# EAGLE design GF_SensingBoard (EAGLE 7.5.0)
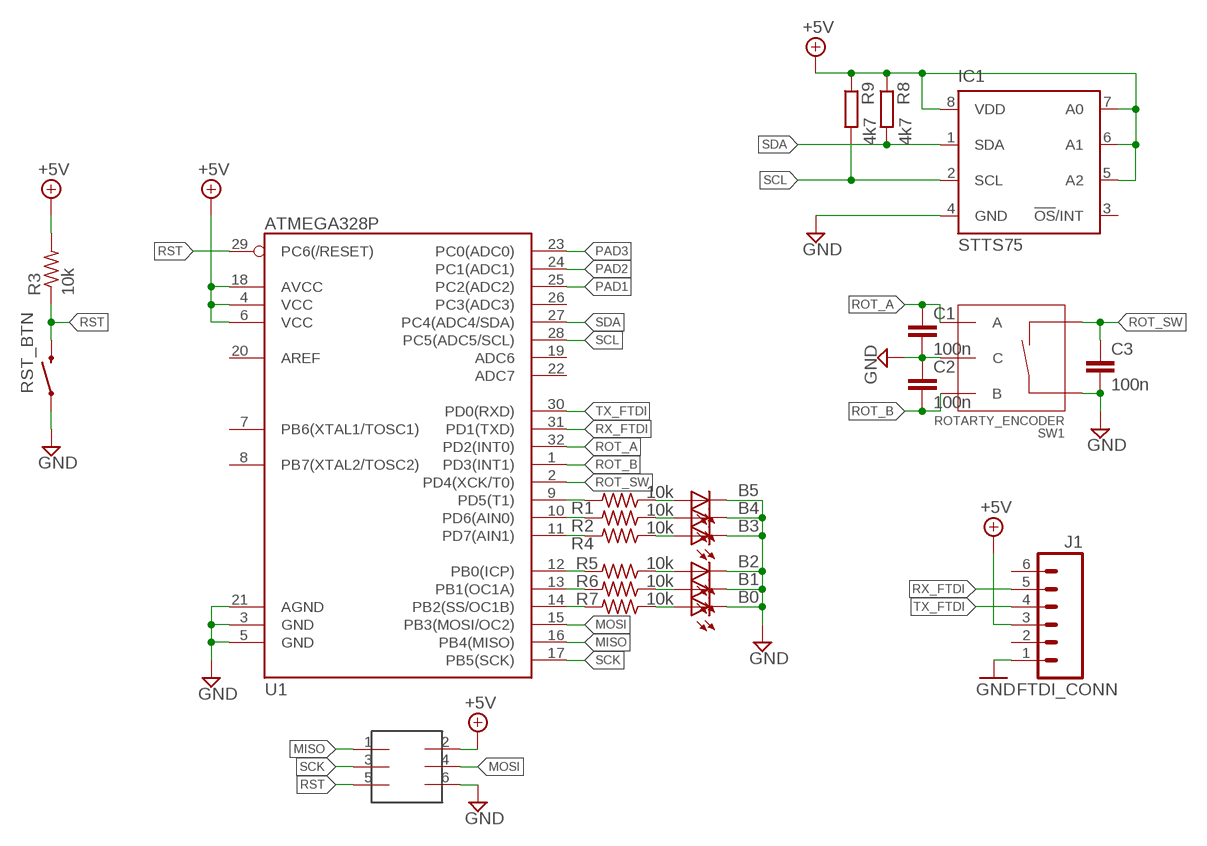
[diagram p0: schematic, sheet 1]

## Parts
B0  LEDCHIPLED_1206  [CHIPLED_1206]
B1  LEDCHIPLED_1206  [CHIPLED_1206]
B2  LEDCHIPLED_1206  [CHIPLED_1206]
B3  LEDCHIPLED_1206  [CHIPLED_1206]
B4  LEDCHIPLED_1206  [CHIPLED_1206]
B5  LEDCHIPLED_1206  [CHIPLED_1206]
C1  100n  C-EUC0603  [C0603]
C2  100n  C-EUC0603  [C0603]
C3  100n  C-EUC0603  [C0603]
IC1  STTS75  [SO08]
ISP  2X3HEADER  [2X3_SMD]
J1  FTDI_CONN  M06SMD  [1X06-SMD]
R1  10k  R-US_R0603  [R0603]
R2  10k  R-US_R0603  [R0603]
R3  10k  R-US_R0603  [R0603]
R4  10k  R-US_R0603  [R0603]
R5  10k  R-US_R0603  [R0603]
R6  10k  R-US_R0603  [R0603]
R7  10k  R-US_R0603  [R0603]
R8  4k7  R-EU_R1206  [R1206]
R9  4k7  R-EU_R1206  [R1206]
RST_BTN  SWITCH2  [TACTILE-SWITCH-1101NE]
SW1  ROTARTY_ENCODER  [ROTARY_ENC_PLAIN]
U1  ATMEGA328P  ATMEGA328_SMT  [TQFP32-08]

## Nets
+5V: IC1.5(A2) IC1.6(A1) IC1.7(A0) IC1.8(VDD) ISP.2 J1.3 R3.2 R8.1 R9.1 U1.4(VCC) U1.6(VCC) U1.18(AVCC)
GND: B0.C B1.C B2.C B3.C B4.C B5.C C1.2 C2.1 C3.2 IC1.4(GND) ISP.6 J1.1 RST_BTN.P$1 SW1.C SW1.SW+ U1.3(GND) U1.5(GND) U1.21(AGND)
MISO: ISP.1 U1.16(PB4(MISO))
MOSI: ISP.4 U1.15(PB3(MOSI/OC2))
N$1: R1.2 U1.9(PD5(T1))
N$2: R2.2 U1.10(PD6(AIN0))
N$3: R4.2 U1.11(PD7(AIN1))
N$4: R5.2 U1.12(PB0(ICP))
N$5: R6.2 U1.13(PB1(OC1A))
N$6: R7.2 U1.14(PB2(SS/OC1B))
N$7: B5.A R1.1
N$8: B4.A R2.1
N$9: B3.A R4.1
N$10: B2.A R5.1
N$11: B1.A R6.1
N$12: B0.A R7.1
PAD1: U1.25(PC2(ADC2))
PAD2: U1.24(PC1(ADC1))
PAD3: U1.23(PC0(ADC0))
ROT_A: C1.1 SW1.A U1.32(PD2(INT0))
ROT_B: C2.2 SW1.B U1.1(PD3(INT1))
ROT_SW: C3.1 SW1.SW- U1.2(PD4(XCK/T0))
RST: ISP.5 R3.1 RST_BTN.P$2 U1.29(PC6(/RESET))
RX_FTDI: J1.5 U1.31(PD1(TXD))
SCK: ISP.3 U1.17(PB5(SCK))
SCL: IC1.2(SCL) R9.2 U1.28(PC5(ADC5/SCL))
SDA: IC1.1(SDA) R8.2 U1.27(PC4(ADC4/SDA))
TX_FTDI: J1.4 U1.30(PD0(RXD))
Unconnected: IC1.3(!OS!/INT) J1.2 J1.6 U1.7(PB6(XTAL1/TOSC1)) U1.8(PB7(XTAL2/TOSC2)) U1.19(ADC6) U1.20(AREF) U1.22(ADC7) U1.26(PC3(ADC3))

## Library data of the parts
B0 B1-B5 = led:LED: LED
C1-C3 = rcl:C-EU: CAPACITOR, European symbol
IC1 = st-micro-add:STTS75: General purpose bipolar Timer
ISP = mellis:2X3HEADER
J1 = SparkFun-Connectors:M06: Header 6 Standard 6-pin 0.1" header. Use with straight break away headers (SKU : PRT-00116), right angle break away headers (PRT-00553), swiss pins (PRT-00743), machine pins (PRT-00117), and female headers (PRT-00115). Molex polarized connector foot print use with SKU : PRT-08094 with associated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; PROD_ID: CONN-08971; VALUE: RA 6Pin SMD
R1-R7 = rcl:R-US_: RESISTOR, American symbol
R8 R9 = rcl:R-EU_: RESISTOR, European symbol
RST_BTN = SparkFun-Electromechanical_2:SWITCH2
SW1 = SparkFun-Electromechanical_2:ROTARTY_ENCODER: Simple no LED rotary encoder Example: COM-09117
U1 = SparkFun-DigitalIC:ATMEGA328_SMT: 32-Pin Atmega328 part Commonly used on Arduino compatible boards Available in QFP and QFN packages TQFP is IC-09069 QFN is non-stock; PROD_ID: IC-09069

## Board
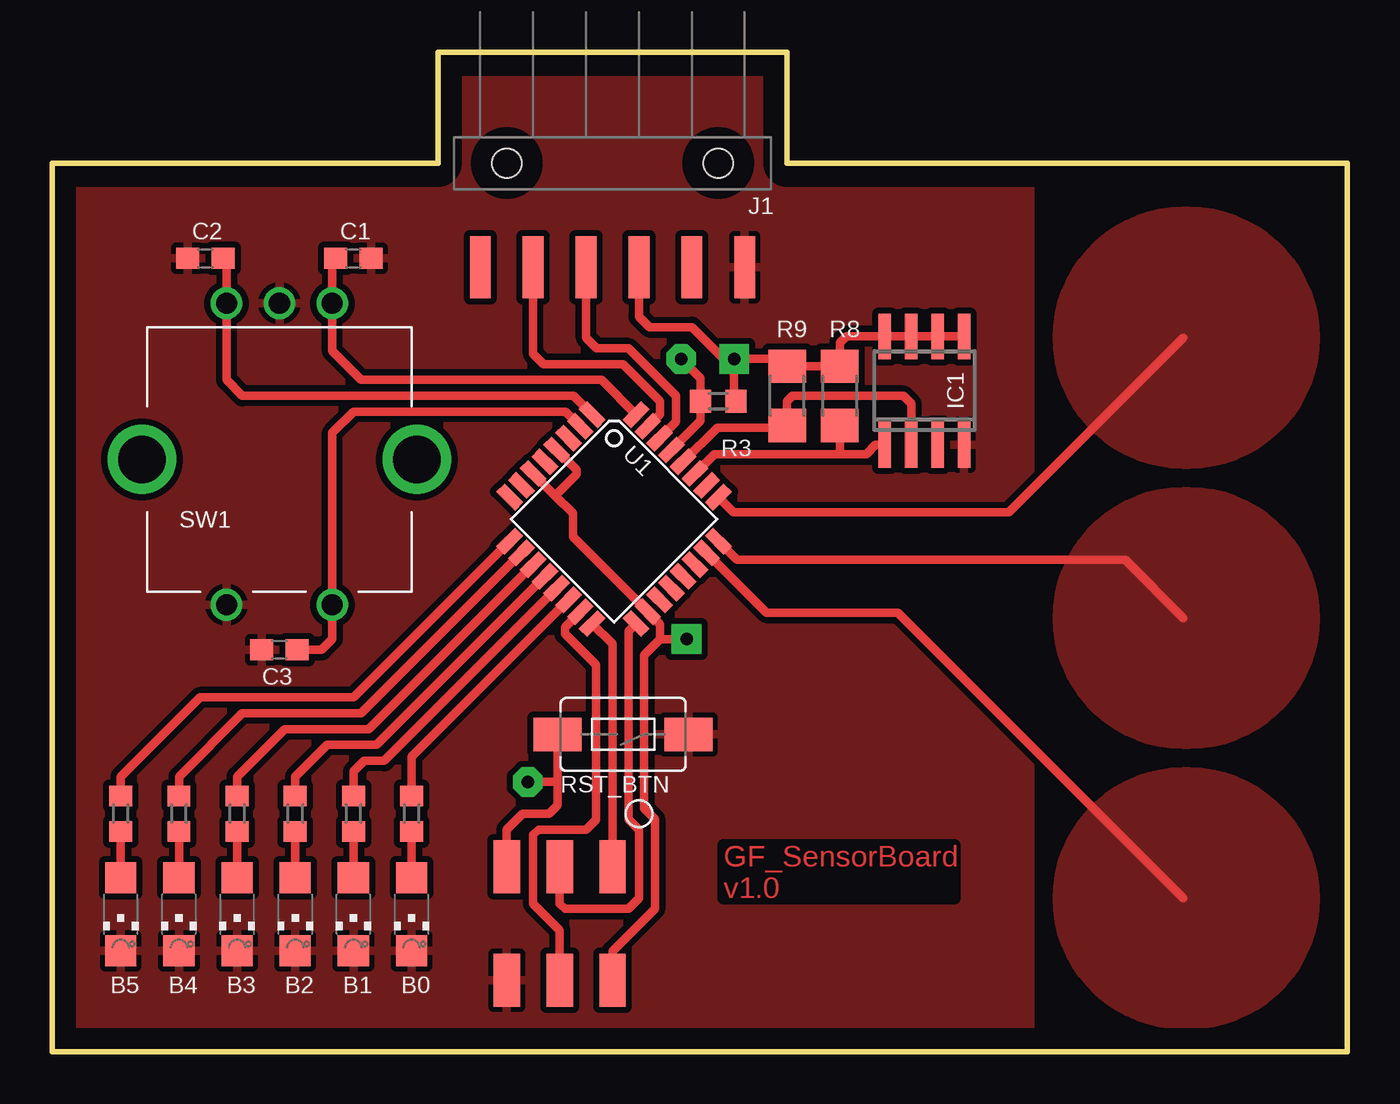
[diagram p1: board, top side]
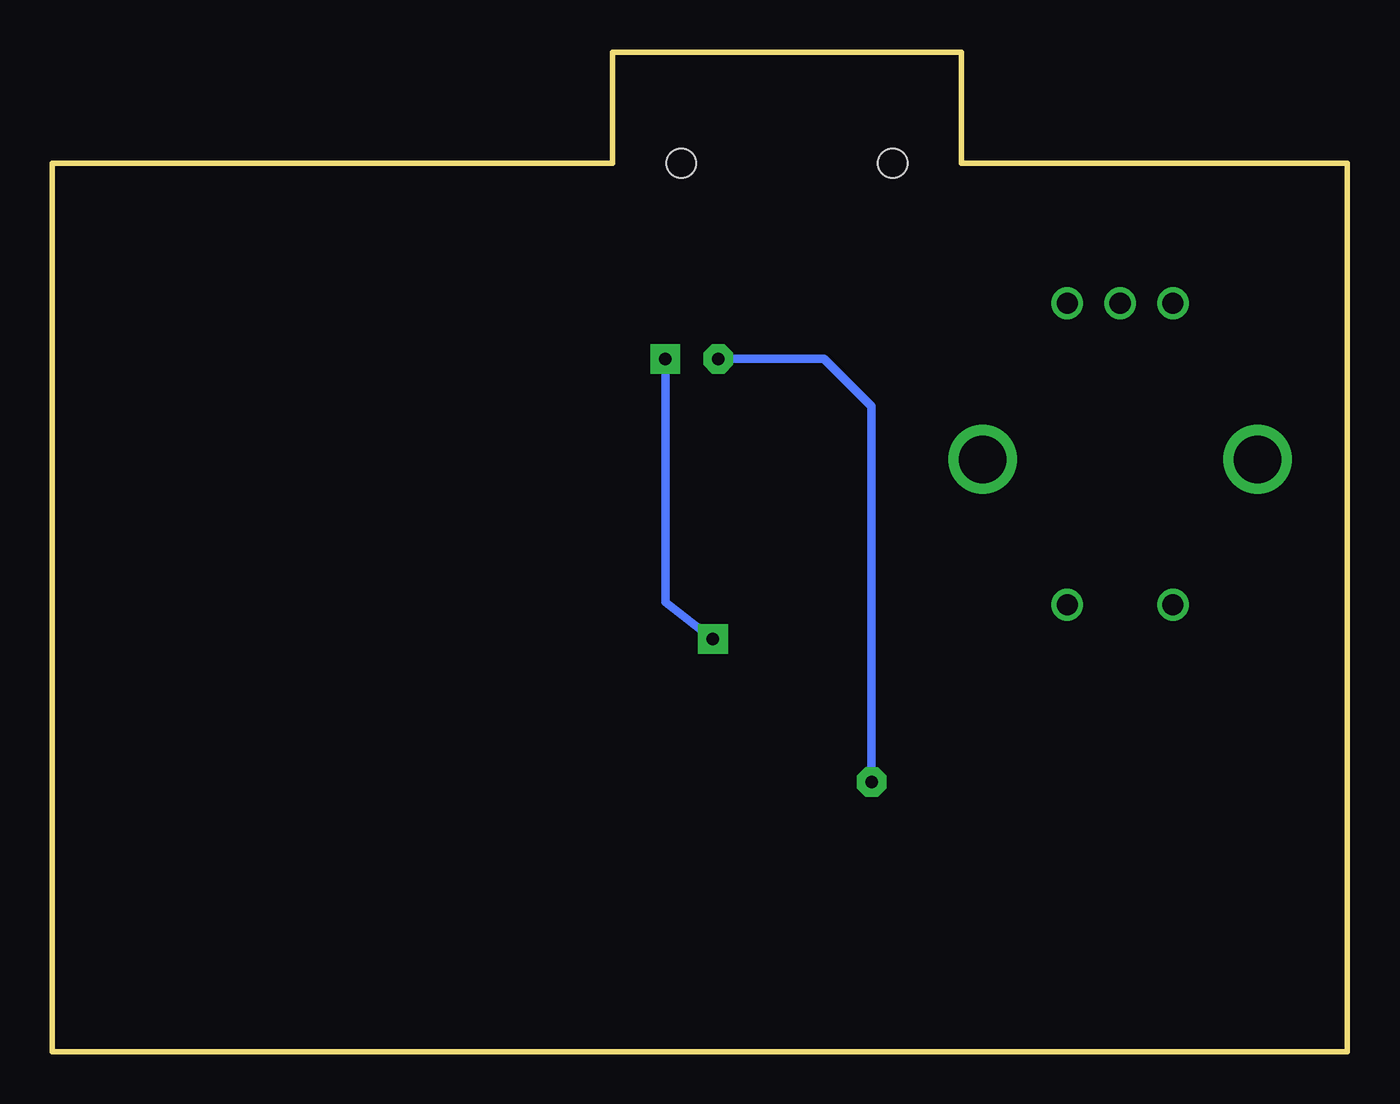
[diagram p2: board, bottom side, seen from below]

Size 62.23 x 48.01 mm. Coordinates in mm from the lower left corner, seen from the top.
Outline: 35.31,42.67 35.31,48.01 18.54,48.01 18.54,42.67 0,42.67 0,0 62.23,0 62.23,42.67 35.31,42.67
Copper layers (1*16): Top 0.035mm / dielectric 1.5mm / Bottom 0.035mm
Design rules "default *": minimum track width 10mil, minimum drill 20mil, track to track 8mil, track to pad 8mil, pad to pad 9.5mil, via to via 8mil, smd to smd 8mil, copper to edge 40mil, drill to drill 8mil, minimum pad ring 10mil, minimum via ring 8mil, stop-mask expansion 4mil, vias tented up to drill 0mil, thermal gap 10mil

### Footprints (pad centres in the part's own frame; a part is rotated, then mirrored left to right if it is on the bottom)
CHIPLED_1206 = smd 1.5 x 1.5: A 0,-1.75; C 0,1.75
C0603 = smd 1.1 x 1: 1 -0.85,0; 2 0.85,0
SO08 = smd 0.6 x 2.2: 1 -1.905,-2.6; 2 -0.635,-2.6; 3 0.635,-2.6; 4 1.905,-2.6; 5 1.905,2.6; 6 0.635,2.6; 7 -0.635,2.6; 8 -1.905,2.6
2X3_SMD = smd 2.54 x 1.27: 1 -2.54,2.54; 2 2.92,2.54; 3 -2.54,0; 4 2.92,0; 5 -2.54,-2.54; 6 2.92,-2.54
1X06-SMD = smd 1 x 3: 1 -6.35,5; 2 -3.81,5; 3 -1.27,5; 4 1.27,5; 5 3.81,5; 6 6.35,5 | hole 1.4: -5.08,0; 5.08,0
R0603 = smd 1 x 1.1: 1 -0.85,0; 2 0.85,0
R1206 = smd 1.6 x 1.803: 1 -1.422,0; 2 1.422,0
TACTILE-SWITCH-1101NE = smd 2.3 x 1.6: P$1 -3.15,0; P$2 3.15,0
ROTARY_ENC_PLAIN = drill 1.016: A 7.493,-2.54; B 7.493,2.54; C 7.493,0; SW+ -6.985,2.54; SW- -6.985,-2.54 | drill 2.286: P$3 0,6.604; P$4 0,-6.604
TQFP32-08 = smd 1.27 x 0.559: 1 -4.293,2.8; 2 -4.293,2; 3 -4.293,1.2; 4 -4.293,0.4; 5 -4.293,-0.4; 6 -4.293,-1.2; 7 -4.293,-2; 8 -4.293,-2.8; 17 4.293,-2.8; 18 4.293,-2; 19 4.293,-1.2; 20 4.293,-0.4; 21 4.293,0.4; 22 4.293,1.2; 23 4.293,2; 24 4.293,2.8 | smd 0.559 x 1.27: 9 -2.8,-4.293; 10 -2,-4.293; 11 -1.2,-4.293; 12 -0.4,-4.293; 13 0.4,-4.293; 14 1.2,-4.293; 15 2,-4.293; 16 2.8,-4.293; 25 2.8,4.293; 26 2,4.293; 27 1.2,4.293; 28 0.4,4.293; 29 -0.4,4.293; 30 -1.2,4.293; 31 -2,4.293; 32 -2.8,4.293

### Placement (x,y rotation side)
B0  17.27,6.6 180 top
B1  14.48,6.6 180 top
B2  11.68,6.6 180 top
B3  8.89,6.6 180 top
B4  6.1,6.6 180 top
B5  3.3,6.6 180 top
C1  14.48,38.1 0 top
C2  7.37,38.1 0 top
C3  10.92,19.3 180 top
IC1  41.91,31.75 0 top
ISP  24.38,6.35 270 top
J1  26.92,42.67 180 top
R1  3.3,11.43 90 top
R2  6.1,11.43 90 top
R3  32,31.24 0 top
R4  8.89,11.43 90 top
R5  11.68,11.43 90 top
R6  14.48,11.43 90 top
R7  17.27,11.43 90 top
R8  37.85,31.5 270 top
R9  35.31,31.5 270 top
RST_BTN  27.43,15.24 180 top
SW1  10.92,28.45 90 top
U1  27,25.58 315 top

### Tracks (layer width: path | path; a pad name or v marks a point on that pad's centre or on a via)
+5V  (via drill 0.6 pad 1.42)
  Top 0.406: U1.6 24.17,26.71 | 24.17,26.71 25.02,25.86 25.02,24.73 U1.18 29.21,20.54 29.21,19.81 | U1.4 25.2,27.94 25.2,27.73 24.17,26.71 | ISP.2 26.92,4.83 28.96,6.86 28.96,11.18 28.45,11.68 28.45,19.05 29.21,19.81 | J1.3 28.19,35.31 28.7,34.8 30.73,34.8 32.26,33.27 v32.77,33.27 | R3.2 32.77,31.33 v32.77,33.27 | 29.21,19.81 v30.48,19.81 | IC1.5 IC1.6 IC1.7 IC1.8 38.16,34.35 37.85,34.04 R8.1 R9.1 34.95,33.27 v32.77,33.27
  Bottom 0.406: v32.77,33.27 32.77,21.59 v30.48,19.81
GND
  pour Top (isolate 0.305, rank 2): 0,0 46.99,0 46.99,42.67 35.31,42.67 35.31,48.01 18.54,48.01 18.54,42.67 0,42.67
MISO
  Top 0.406: ISP.1 26.92,19.58 U1.16
MOSI
  Top 0.406: ISP.4 24.38,5.84 23.11,7.11 23.11,10.41 23.37,10.67 25.65,10.67 26.13,11.14 26.13,18.57 24.64,20.07 24.64,20.39 U1.15
N$1
  Top 0.406: U1.9 14.48,17.02 7.11,17.02 3.3,13.21 R1.2
N$2
  Top 0.406: U1.10 14.85,16.26 9.14,16.26 6.1,13.21 R2.2
N$3
  Top 0.406: U1.11 15.22,15.49 11.18,15.49 8.89,13.21 R4.2
N$4
  Top 0.406: U1.12 15.59,14.73 13.21,14.73 11.68,13.21 R5.2
N$5
  Top 0.406: U1.13 15.95,13.97 14.99,13.97 14.48,13.46 R6.2
N$6
  Top 0.406: U1.14 17.27,14.16 R7.2
N$7
  Top 0.406: R1.1 B5.A
N$8
  Top 0.406: R2.1 B4.A
N$9
  Top 0.406: R4.1 B3.A
N$10
  Top 0.406: R5.1 B2.A
N$11
  Top 0.406: R6.1 B1.A
N$12
  Top 0.406: R7.1 B0.A
PAD1
  Top 0.406: U1.25 32.74,25.91 45.97,25.91 54.36,34.29
  pour Top: 48.26,34.29 arc90 54.36,28.19 54.61,28.19 arc90 60.71,34.29 arc90 54.61,40.39 54.36,40.39 arc90
PAD2
  Top 0.406: U1.24 32.92,23.62 51.56,23.62 54.36,20.83
  pour Top: 48.26,20.83 arc90 54.36,14.73 54.61,14.73 arc90 60.71,20.83 arc90 54.61,26.92 54.36,26.92 arc90
PAD3
  Top 0.406: U1.23 34.32,21.08 40.64,21.08 54.36,7.37
  pour Top: 48.26,7.37 arc90 54.36,1.27 54.61,1.27 arc90 60.71,7.37 arc90 54.61,13.46 54.36,13.46 arc90
ROT_A
  Top 0.406: U1.32 26.39,32.26 14.86,32.26 13.46,33.66 SW1.A 13.46,37.93 C1.1
ROT_B
  Top 0.406: U1.1 25.04,31.5 9.14,31.5 8.38,32.26 SW1.B 8.38,37.93 C2.2
ROT_SW
  Top 0.406: U1.2 24.67,30.73 14.48,30.73 13.46,29.72 SW1.SW- 13.46,19.81 12.95,19.3 C3.1
RST  (via drill 0.6 pad 1.42)
  Top 0.406: U1.29 31.15,30.3 R3.1 31.15,32.35 v30.23,33.27 | RST_BTN.P$2 24.28,12.95 | 24.28,12.95 24.28,11.84 23.88,11.43 22.61,11.43 21.84,10.67 ISP.5 | v22.86,12.95 24.28,12.95
  Bottom 0.406: v22.86,12.95 22.86,30.99 25.15,33.27 v30.23,33.27
RX_FTDI
  Top 0.406: U1.31 29.21,30.62 29.21,31.24 27.43,33.02 23.62,33.02 23.11,33.53 J1.5
SCK
  Top 0.406: ISP.3 24.38,7.11 24.64,6.86 27.69,6.86 28.19,7.37 28.19,10.67 27.69,11.18 27.69,20.2 U1.17
SCL
  Top 0.406: U1.28 31.96,29.97 35.2,29.97 R9.2 35.31,31.24 35.56,31.5 40.89,31.5 41.27,31.11 IC1.2
SDA
  Top 0.406: U1.27 31.82,28.7 37.85,28.7 | 37.85,28.7 39.12,28.7 39.56,29.15 IC1.1 | R8.2 37.85,28.7
TX_FTDI
  Top 0.406: U1.30 29.97,30.25 29.97,31.5 27.69,33.78 26.16,33.78 25.65,34.29 J1.4

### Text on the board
Top: GF_SensorBoard / v1.0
